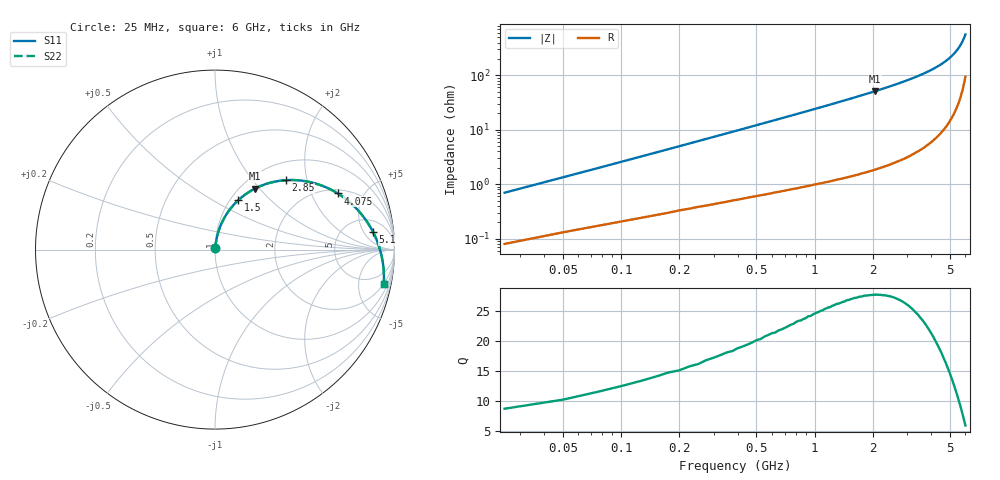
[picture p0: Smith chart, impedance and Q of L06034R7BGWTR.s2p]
!	AVX Thin Film Operation
!	Date:	March	2003
!	Description: Accu-L® Series Thin Film SMD RF Inductors
!	Part Number: L06034R7BGWTR
!	25MHz-6GHz
!	Serial	Measurements
#	mhz	S	db	R	50
!	S11	S11	S21	S21	S12	S12	S22	S22
!	dB	Phase	dB	Phase	dB	Phase	dB	Phase
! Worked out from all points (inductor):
!   240 points, 25 MHz to 6 GHz, reference 50 ohm
!   read as one part in series: L = 4.13 nH near 50 MHz
!   highest Q = 27.7 at 2.05 GHz (marker M1), where L = 3.97 nH
!   S11 on the Smith chart (normalised r, x): 25 MHz: 1.00, +0.01; 1.5 GHz: 1.09, +0.66; 2.85 GHz: 1.35, +1.50; 4.075 GHz: 2.20, +3.17; 5.1 GHz: 9, +8; 6 GHz: 2.02, -9.61
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25  -44.08 82.1  -0.01 -0.4  -0.01 -0.4  -44.08 82.1
50  -38.51 82.9  -0.01 -0.8  -0.01 -0.8  -38.51 82.9
75  -35.21 83.1  -0.02 -1.2  -0.02 -1.2  -35.21 83.1
100  -32.86 83.2  -0.02 -1.6  -0.02 -1.6  -32.86 83.2
175  -28.25 82.8  -0.03 -2.8  -0.03 -2.8  -28.25 82.8
275  -24.51 81.8  -0.05 -4.3  -0.05 -4.3  -24.51 81.8
400  -21.39 80.3  -0.08 -6.2  -0.08 -6.2  -21.39 80.3
575  -18.37 78.0  -0.12 -8.8  -0.12 -8.8  -18.37 78.0
775  -15.87 75.3  -0.18 -11.8  -0.18 -11.8  -15.87 75.3
1025  -13.54 71.7  -0.28 -15.5  -0.28 -15.5  -13.54 71.7
1500  -10.37 64.9  -0.53 -22.6  -0.53 -22.6  -10.37 64.9
2025  -7.91 57.1  -0.91 -30.5  -0.91 -30.5  -7.91 57.1
2050  -7.80 56.7  -0.93 -30.8  -0.93 -30.8  -7.80 56.7
2850  -5.16 44.5  -1.79 -43.0  -1.79 -43.0  -5.16 44.5
3025  -4.69 41.7  -2.03 -45.7  -2.03 -45.7  -4.69 41.7
3525  -3.52 33.7  -2.86 -53.5  -2.86 -53.5  -3.52 33.7
4025  -2.56 25.4  -3.93 -61.5  -3.93 -61.5  -2.56 25.4
4075  -2.47 24.5  -4.06 -62.3  -4.06 -62.3  -2.47 24.5
5025  -1.13 7.7  -7.38 -78.0  -7.38 -78.0  -1.13 7.7
5100  -1.05 6.3  -7.76 -79.2  -7.76 -79.2  -1.05 6.3
5625  -0.58 -3.8  -11.22 -87.4  -11.22 -87.4  -0.58 -3.8
6000  -0.36 -11.4  -15.40 -91.5  -15.40 -91.5  -0.36 -11.4
